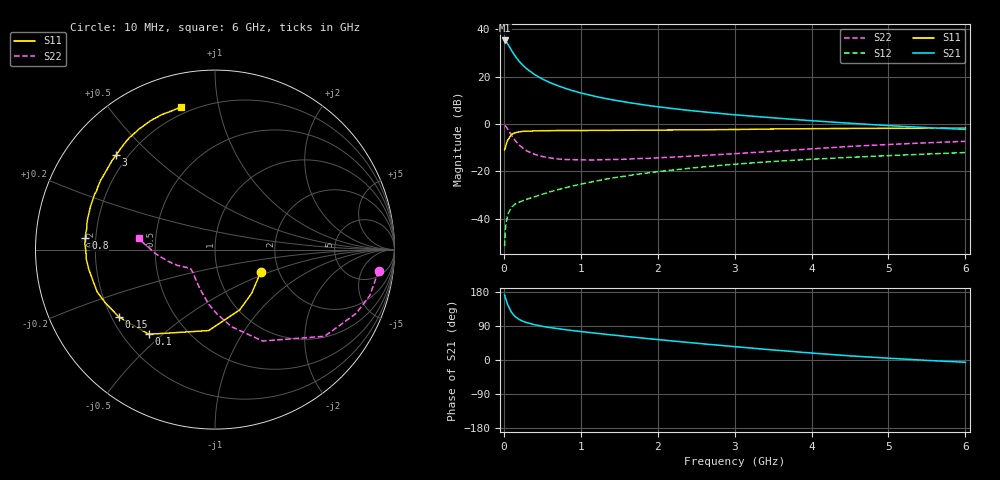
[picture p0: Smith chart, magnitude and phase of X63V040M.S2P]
! SIEMENS Small Signal Semiconductors
! BFP193W
! Si NPN RF Bipolar Junction Transistor in SOT343
! VCE = 3 V  IC = 40 mA
! Common Emitter S-Parameters:  April 1994
# GHz  S  MA  R  50
!  f  S11  S21  S12  S22
! GHz  MAG  ANG  MAG  ANG  MAG  ANG  MAG  ANG
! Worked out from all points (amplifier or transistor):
!   40 points, 10 MHz to 6 GHz, reference 50 ohm
!   highest |S21| = 35.3 dB at 10 MHz (marker M1)
!   |S21| within 3 dB of that: start of sweep to 78.25 MHz
!   unconditionally stable (mu >= 1): 670.7 MHz to 3.998 GHz
!   at 200 MHz: K = 0.53, MSG = 29.8 dB, |S12| = -33.1 dB
!   at 1.5 GHz: K = 1.13, MAG = 13.9 dB, |S12| = -22.4 dB
!   at 6 GHz: K = 0.94, MSG = 4.9 dB, |S12| = -12.1 dB
!   S11 on the Smith chart (normalised r, x): 10 MHz: 1.61, -0.44; 100 MHz: 0.31, -0.45; 150 MHz: 0.23, -0.30; 800 MHz: 0.16, +0.04; 3 GHz: 0.16, +0.39; 6 GHz: 0.16, +0.77
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0.01  0.2836 -26.4  58.24 171.6  0.0026 86.8  0.9194 -7.4
0.02  0.3175 -49.8  57.06 165.0  0.0056 74.9  0.8996 -16.6
0.03  0.3631 -67.7  55.11 158.0  0.008 72.1  0.8627 -24.4
0.05  0.4526 -94.5  49.38 145.8  0.012 61.9  0.7788 -38.3
0.1  0.5986 -128.0  35.89 125.6  0.0174 49.2  0.5749 -62.4
0.15  0.6533 -144.9  26.81 113.9  0.0204 44.2  0.4397 -77.9
0.2  0.6803 -154.4  21.02 106.9  0.0222 44.6  0.3576 -88.4
0.25  0.6973 -160.3  17.27 102.1  0.0239 44.6  0.3068 -96.4
0.3  0.7009 -165.0  14.52 98.6  0.0256 46.2  0.2683 -102.9
0.4  0.7121 -171.3  11.06 93.1  0.0288 49.4  0.2272 -112.8
0.5  0.7191 -175.8  8.929 89.0  0.0326 52.1  0.2049 -120.2
0.6  0.7196 -179.4  7.463 85.6  0.0366 54.5  0.1906 -126.0
0.8  0.7247 174.9  5.639 80.0  0.0446 58.1  0.1769 -133.3
1.1  0.7284 168.5  4.137 72.9  0.0575 60.2  0.1728 -140.3
1.3  0.7306 164.5  3.506 68.4  0.0667 60.9  0.1755 -142.7
1.6  0.7348 158.9  2.873 62.0  0.0798 60.5  0.1797 -145.6
2.2  0.745 148.9  2.112 50.1  0.1062 58.1  0.1987 -151.4
3  0.7619 136.3  1.561 35.3  0.1404 53.0  0.2344 -159.3
3.2  0.7693 133.3  1.471 31.8  0.1486 51.5  0.2463 -161.3
4.5  0.8031 116.4  1.034 10.9  0.1966 42.0  0.3347 -176.4
5.5  0.809 107.8  0.835 -1.0  0.2307 35.3  0.3988 174.9
6  0.8161 103.6  0.766 -6.0  0.2484 32.3  0.4288 171.7
